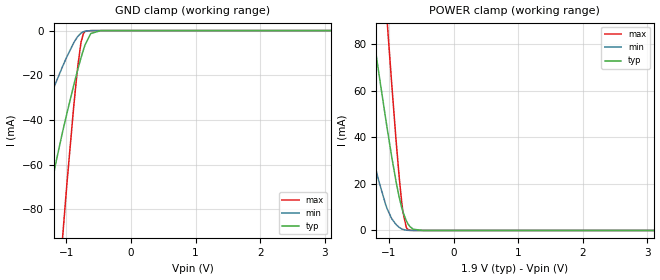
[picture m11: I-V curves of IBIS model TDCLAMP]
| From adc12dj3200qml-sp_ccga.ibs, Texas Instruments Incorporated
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[Model]   TDCLAMP
Model_type   Terminator
|   typ   min   max
C_comp   0.55pF   0.47pF   0.62pF
[Voltage Range]   1.9   1.8   2
[Temperature Range]   25   125   -40
[Power Clamp Reference]   1.9   1.8   2
[GND Clamp Reference]   0   0   0
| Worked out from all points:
|   GND clamp passes 1 mA (typ) near -0.59 V on its own axis
|   POWER clamp passes 1 mA (typ) near -0.65 V on its own axis
[GND Clamp]
|   Voltage   I(typ)   I(min)   I(max)
-1.9V     -241.5mA   -111.9mA   -561.3mA
-1.575V   -152.4mA   -60.14mA   -369.8mA
-1.359V   -96.95mA   -37.61mA   -244.7mA
-1.313V   -86.43mA   -34.13mA   -219mA
-1.205V   -65.32mA   -26.2mA    -159.9mA
-1.056V   -44.88mA   -15.84mA   -91.34mA
-839.8mV  -19.1mA    -3.239mA   -20.15mA
-777.1mV  -12.44mA   -1.195mA   -5.778mA
-737.2mV  -8.617mA   -514.4uA   -1.347mA
-623.2mV  -1.309mA   -28.37uA   -4.292uA
-469.3mV  -14.31uA   -455.5nA   0A
3.8V      0A         0A         0A
[POWER Clamp]
|   Voltage   I(typ)   I(min)   I(max)
-1.9V     214.2mA    115.2mA    444.3mA
-1.467V   127.6mA    58.41mA    265.8mA
-1.33V    100.8mA    41.3mA     210.1mA
-1.227V   81mA       29.07mA    168.7mA
-1.028V   43.95mA    9.338mA    89.85mA
-965.2mV  33.07mA    5.512mA    66.04mA
-879.7mV  19.55mA    2.266mA    35.38mA
-799.9mV  9.59mA     638.4uA    11.59mA
-731.5mV  4.195mA    136uA      1.401mA
-674.5mV  1.647mA    31.47uA    96.06uA
-469.3mV  5.252uA    129.6nA    761.5pA
3.8V      0A         0A         0A
